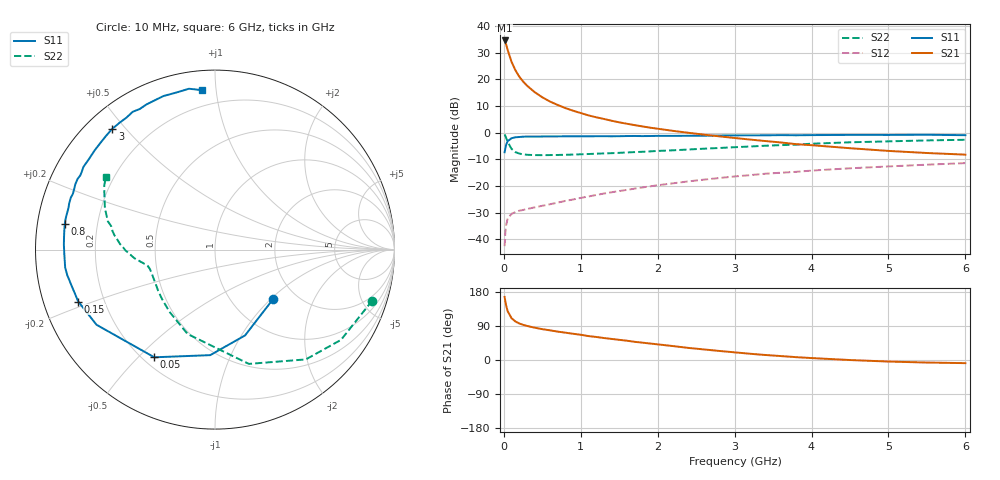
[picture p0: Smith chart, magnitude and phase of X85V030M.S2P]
! SIEMENS Small Signal Semiconductors
! BFP136W
! Si NPN RF Bipolar Junction Transistor in SOT343
! VCE = 5 V  IC = 30 mA
! Common Emitter S-Parameters:  September  1994
# GHz  S  MA  R  50
!  f  S11  S21  S12  S22
! GHz  MAG  ANG  MAG  ANG  MAG  ANG  MAG  ANG
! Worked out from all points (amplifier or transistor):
!   40 points, 10 MHz to 6 GHz, reference 50 ohm
!   highest |S21| = 34.5 dB at 10 MHz (marker M1)
!   |S21| within 3 dB of that: start of sweep to 44.2 MHz
!   unconditionally stable (mu >= 1): 833.3 MHz to 2.815 GHz
!   at 200 MHz: K = 0.42, MSG = 25.1 dB, |S12| = -29.3 dB
!   at 1.5 GHz: K = 1.14, MAG = 10.6 dB, |S12| = -21.9 dB
!   at 6 GHz: K = 0.96, MSG = 1.6 dB, |S12| = -11.5 dB
!   S11 on the Smith chart (normalised r, x): 10 MHz: 1.54, -1.03; 50 MHz: 0.24, -0.56; 150 MHz: 0.11, -0.18; 800 MHz: 0.08, +0.08; 3 GHz: 0.08, +0.46; 6 GHz: 0.11, +0.92
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0.01  0.4253 -40.2  53.23 166.4  0.0074 75.2  0.9208 -18.0
0.02  0.5066 -70.7  48.97 153.9  0.0138 66.4  0.8636 -35.6
0.03  0.5887 -92.6  44.62 143.7  0.0183 56.3  0.7939 -50.4
0.05  0.6887 -119.4  35.17 128.6  0.0245 44.2  0.6642 -73.5
0.1  0.7817 -147.6  21.19 110.3  0.0299 31.7  0.4943 -108.0
0.15  0.8149 -159.2  14.76 101.7  0.0322 29.2  0.4295 -126.2
0.2  0.8237 -165.7  11.19 96.5  0.0342 28.0  0.4033 -137.2
0.25  0.8354 -170.2  9.056 92.8  0.0353 29.3  0.3908 -144.3
0.3  0.8408 -173.1  7.593 90.0  0.0368 30.2  0.3825 -149.4
0.4  0.8399 -178.2  5.726 85.3  0.0395 33.5  0.3776 -155.8
0.5  0.8424 178.2  4.574 81.4  0.0423 36.3  0.3764 -159.9
0.6  0.8438 175.5  3.81 78.3  0.0452 39.2  0.3778 -162.3
0.7  0.8463 172.8  3.285 74.9  0.0485 41.9  0.3794 -163.9
0.8  0.8489 170.4  2.873 72.1  0.0522 43.9  0.3829 -165.3
1.1  0.8487 164.0  2.096 63.1  0.0632 48.6  0.3954 -167.9
1.5  0.8529 157.1  1.553 53.2  0.08 52.1  0.4163 -170.3
2.2  0.8647 144.4  1.074 36.7  0.1117 52.1  0.4642 -175.5
3  0.8833 130.4  0.79 20.2  0.15 47.8  0.5304 176.6
3.2  0.8845 127.0  0.738 16.5  0.1588 46.3  0.5467 174.2
4.5  0.9025 108.6  0.508 -0.1  0.2135 35.3  0.6553 159.4
5.5  0.9079 99.2  0.413 -6.7  0.2496 27.3  0.7113 150.2
6  0.8915 94.7  0.385 -8.3  0.267 22.9  0.7311 146.4
